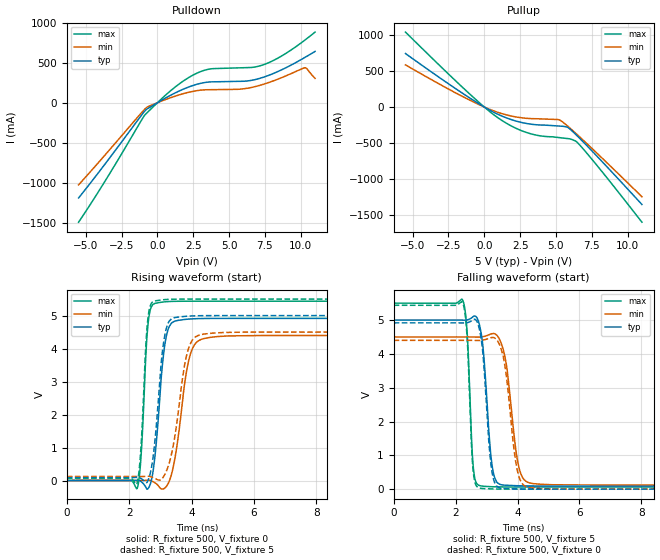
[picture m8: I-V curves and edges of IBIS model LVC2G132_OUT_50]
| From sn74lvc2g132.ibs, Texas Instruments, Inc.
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[Model]   LVC2G132_OUT_50
Model_type  Output
Vref =   0
Rref =   500
Cref =   50p
Vmeas =   2.5
| variable   typ   min   max
C_comp   8.96pF   5.47pF   12.37pF
| C_pullup   9.70pF   5.47pF   12.37pF
| C_pulldown   8.22pF   6.21pF   11.62pF
[Temperature Range]   40   100   -40
| Ambient temperature   25   85   -40
[Voltage range]   5   4.5   5.5
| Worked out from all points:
|   slope of the pulldown table from 0 to 0.75 V, typ, clamps not added: 9.73 ohm
|   slope of the pullup table from 0 to 0.75 V, typ, clamps not added: 9.16 ohm
|   rising waveform, R_fixture 500, V_fixture 0: 20-80 % time 263ps typ, 378ps min, 166ps max; typ from 0 V to 4.91 V
|   falling waveform, R_fixture 500, V_fixture 5: 20-80 % time 229ps typ, 323ps min, 146ps max; typ from 5 V to 0.091 V
|   rising waveform, R_fixture 500, V_fixture 5: 20-80 % time 269ps typ, 403ps min, 168ps max; typ from 0.091 V to 5 V
|   falling waveform, R_fixture 500, V_fixture 0: 20-80 % time 225ps typ, 318ps min, 145ps max; typ from 4.92 V to 0 V
[Pulldown]
| LVC2G132_OUT_50
|   Voltage   I(typ)   I(min)   I(max)
-5.5V     -1.19A     -1.026A    -1.493A
-3.615V   -756.5mA   -644.9mA   -968mA
-860mV    -99.61mA   -76.72mA   -149.6mA
1.145V    114mA      76.72mA    182.7mA
2.335V    206.5mA    136.8mA    330.4mA
3.39V     254.8mA    162mA      411mA
5.9V      268mA      171.6mA    436.9mA
6.79V     288.1mA    200.2mA    446mA
7.59V     330.6mA    241.7mA    487.6mA
8.82V     424.5mA    324.7mA    600.5mA
10.29V    565.4mA    436.9mA    781.9mA
11V       641.1mA    304.6mA    882.6mA
[Pullup]
| LVC2G132_OUT_50
|   Voltage   I(typ)   I(min)   I(max)
-5.5V     745.2mA    587.5mA    1.044A
-1.18V    147.6mA    112.6mA    211.7mA
1.04V     -109.2mA   -79.97mA   -161.6mA
2.045V    -185.4mA   -131.8mA   -280mA
3.05V     -232.7mA   -158.7mA   -361.3mA
3.945V    -250.5mA   -165.3mA   -402.5mA
5.295V    -265.8mA   -184.8mA   -427.6mA
5.83V     -285.1mA   -267.5mA   -440mA
6.335V    -372.8mA   -357.2mA   -470.5mA
6.54V     -412.8mA   -394.7mA   -503.8mA
8.12V     -739mA     -692.4mA   -876.8mA
11V       -1.358A    -1.25A     -1.605A
[Ramp]
| LVC2G132_OUT_50
| variable   typ   min   max
dV/dt_r   3.10/2.82E-10   2.79/4.08E-10   3.41/1.78E-10
dV/dt_f   3.02/2.42E-10   2.69/3.38E-10   3.34/1.51E-10
R_load = 500
[Rising Waveform]
| LVC2G132_OUT_50
R_fixture =   500
C_fixture =   0
L_fixture =   0
V_fixture =   0
V_fixture_min = 0
V_fixture_max = 0
|   Time   V(typ)   V(min)   V(max)
0s        185.3pV    4.77nV     2.097nV
2.26ns    5.477mV    -233.7uV   -232.4mV
2.385ns   -35.51mV   -347uV     784.2mV
2.615ns   -230.2mV   9.033mV    4.824V
2.935ns   1.887V     -158.7mV   5.39V
3.11ns    3.878V     -248.4mV   5.413V
3.29ns    4.677V     -10.05mV   5.426V
3.94ns    4.895V     3.753V     5.435V
4.585ns   4.912V     4.337V     5.435V
34.99ns   4.914V     4.397V     5.435V
[Falling Waveform]
| LVC2G132_OUT_50
R_fixture =   500
C_fixture =   0
L_fixture =   0
V_fixture =   5
V_fixture_min = 4.5
V_fixture_max = 5.5
|   Time   V(typ)   V(min)   V(max)
0s        5V         4.5V       5.5V
2.235ns   4.998V     4.5V       5.579V
2.38ns    5.006V     4.5V       4.546V
2.575ns   5.108V     4.498V     619.7mV
2.81ns    4.691V     4.499V     97.83mV
3.175ns   731.2mV    4.597V     72.34mV
3.525ns   123.1mV    4.175V     65.81mV
4.03ns    100.8mV    708.8mV    63.54mV
4.495ns   93.99mV    164.8mV    63.05mV
34.99ns   91.34mV    120.7mV    62.83mV
[Rising Waveform]
| LVC2G132_OUT_50
R_fixture =   500
C_fixture =   0
L_fixture =   0
V_fixture =   5
V_fixture_min = 4.5
V_fixture_max = 5.5
|   Time   V(typ)   V(min)   V(max)
0s        91.33mV    120.7mV    62.82mV
2.245ns   95.53mV    120.5mV    -108.9mV
2.375ns   64.94mV    120.3mV    952.9mV
2.595ns   -16mV      129.9mV    4.852V
2.87ns    1.648V     42.15mV    5.451V
3.06ns    3.856V     60.76mV    5.476V
3.25ns    4.769V     424.8mV    5.49V
3.86ns    4.98V      3.857V     5.499V
4.415ns   4.997V     4.441V     5.5V
34.99ns   5V         4.5V       5.5V
[Falling Waveform]
| LVC2G132_OUT_50
R_fixture =   500
C_fixture =   0
L_fixture =   0
V_fixture =   0
V_fixture_min = 0
V_fixture_max = 0
|   Time   V(typ)   V(min)   V(max)
0s        4.917V     4.401V     5.437V
2.23ns    4.915V     4.401V     5.509V
2.375ns   4.922V     4.401V     4.438V
2.565ns   5.009V     4.399V     569.7mV
2.81ns    4.532V     4.4V       25.52mV
3.15ns    678mV      4.48V      8.621mV
3.455ns   29.37mV    4.189V     3.191mV
3.99ns    8.06mV     571mV      715.1uV
4.41ns    2.555mV    39.05mV    256.2uV
34.99ns   13.5uV     21.29uV    8.36uV
